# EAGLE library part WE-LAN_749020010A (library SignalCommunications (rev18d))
WE-LAN LAN Transformer 10/100 Base T - Compliant with IEEE 802.3, IEEE 802.3af and IEEE 802.3at standards - SMT -- Ethernet -- Power over Ethernet -- 1 Gigabit Ethernet -- Compliant with most IC's for ethernet applications like Intel, AMD, Globespan and Realtek -- Hub, Router, Switch Details see: http://katalog.we-online.de/en/pbs/WE-LAN/749020010A 2016 (C) Würth Elektronik
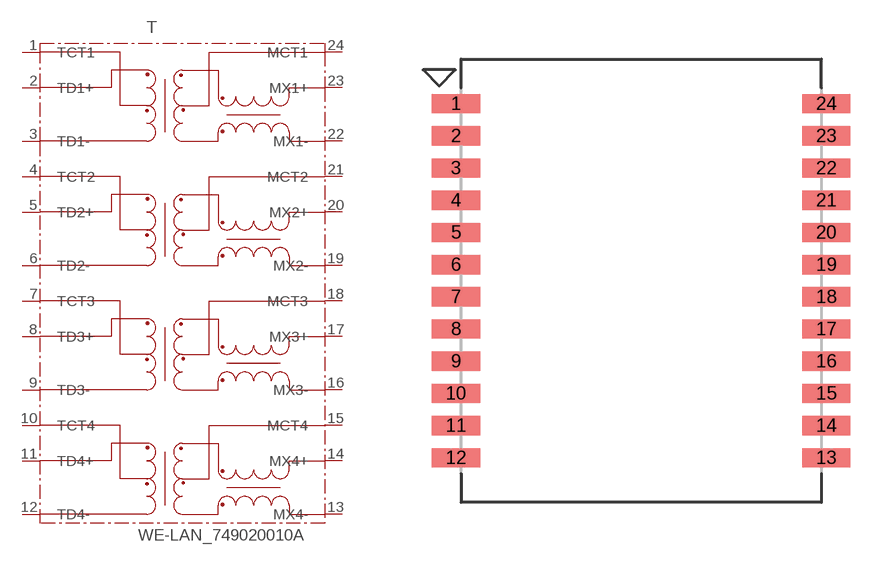
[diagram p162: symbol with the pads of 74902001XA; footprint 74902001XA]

Designator prefix T

## WE-LAN_749020010A  [74902001XA]
1  TCT1
2  TD1+
3  TD1-
4  TCT2
5  TD2+
6  TD2-
7  TCT3
8  TD3+
9  TD3-
10  TCT4
11  TD4+
12  TD4-
13  MX4-
14  MX4+
15  MCT4
16  MX3-
17  MX3+
18  MCT3
19  MX2-
20  MX2+
21  MCT2
22  MX1-
23  MX1+
24  MCT1

## Footprint 74902001XA (pad centres in mm)
smd 1.9 x 0.76: 1 -7.3,6.985; 2 -7.3,5.715; 3 -7.3,4.445; 4 -7.3,3.175; 5 -7.3,1.905; 6 -7.3,0.635; 7 -7.3,-0.635; 8 -7.3,-1.905; 9 -7.3,-3.175; 10 -7.3,-4.445; 11 -7.3,-5.715; 12 -7.3,-6.985; 13 7.3,-6.985; 14 7.3,-5.715; 15 7.3,-4.445; 16 7.3,-3.175; 17 7.3,-1.905; 18 7.3,-0.635; 19 7.3,0.635; 20 7.3,1.905; 21 7.3,3.175; 22 7.3,4.445; 23 7.3,5.715; 24 7.3,6.985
